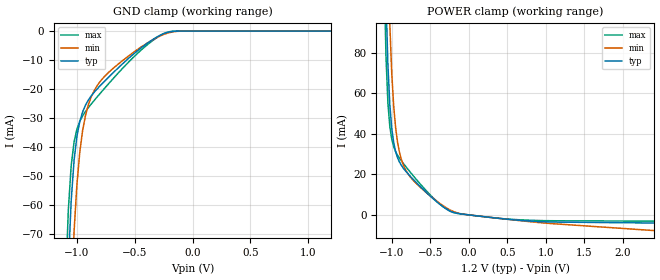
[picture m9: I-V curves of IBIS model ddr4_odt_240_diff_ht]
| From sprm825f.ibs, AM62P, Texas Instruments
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|   Model ddr4_odt_240_diff_ht
[Model] ddr4_odt_240_diff_ht
Model_type Input
Polarity   Non-Inverting
Enable   Active-High
Vinl =  0.700V
Vinh =  0.900V
C_comp   2.860pF   2.855pF   2.930pF
[Model Spec]
Vinh   0.900V   0.820V   0.980V
Vinl   0.700V   0.620V   0.780V
[Temperature Range]   25.000   0.125k   -40.000
[Voltage Range]   1.200V   1.140V   1.260V
[C Comp Corner]
C_comp   2.860pF   2.930pF   2.855pF
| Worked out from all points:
|   GND clamp passes 1 mA (typ) near -0.26 V on its own axis
|   POWER clamp passes 1 mA (typ) near -0.18 V on its own axis
[GND_clamp]
|Voltage   I(typ)   I(min)   I(max)
-1.2V     -394.1mA   -446.5mA   -368.6mA
-1.1V     -116.8mA   -169.3mA   -90.37mA
-1.075V   -81.66mA   -126mA     -62.18mA
-1.05V    -58.74mA   -93.1mA    -46.59mA
-1.025V   -44.71mA   -69.35mA   -38.37mA
-1V       -36.31mA   -52.86mA   -33.86mA
-975mV    -31.18mA   -41.66mA   -31.11mA
-925mV    -25.51mA   -28.94mA   -27.7mA
-800mV    -18.91mA   -17.47mA   -21.58mA
-500mV    -7.591mA   -7.036mA   -8.606mA
-175mV    -128.2uA   -306.4uA   -83.79uA
1.2V      0A         0A         0A
[POWER_clamp]
|Voltage   I(typ)   I(min)   I(max)
-1.2V     595.8mA    733.9mA    624mA
-1.1V     158.8mA    249.7mA    122.2mA
-1.075V   107.2mA    180.5mA    78.56mA
-1.05V    74.3mA     129.8mA    55.44mA
-1.025V   54.44mA    94.17mA    43.64mA
-975mV    35.7mA     53.88mA    33.69mA
-925mV    28.29mA    35.94mA    29.46mA
-875mV    24.44mA    27.38mA    26.67mA
-775mV    19.72mA    19.5mA     21.83mA
-300mV    3.184mA    3.707mA    3.097mA
750mV     -2.951mA   -3.186mA   -2.567mA
2.4V      -4.008mA   -7.726mA   -3.088mA
